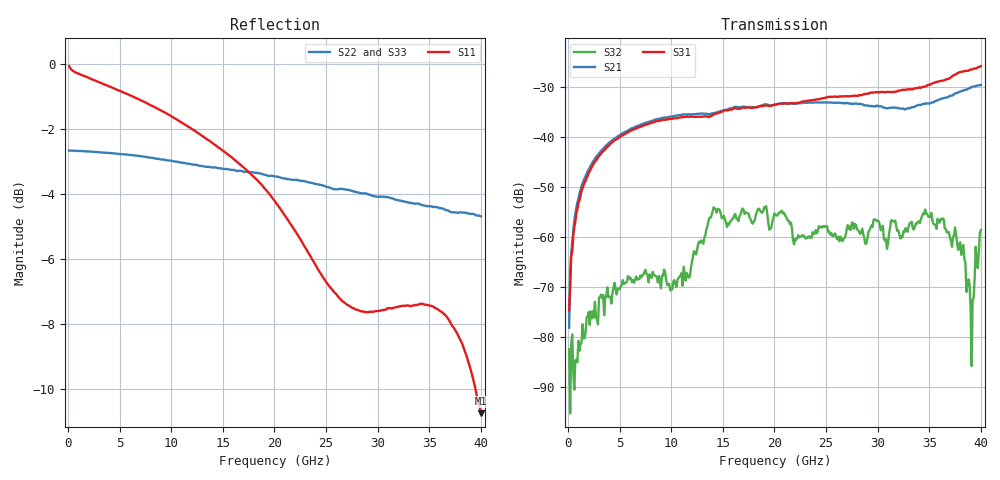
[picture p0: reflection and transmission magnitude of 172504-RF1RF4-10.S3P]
!  3-Port S-parameters saved by WinCal
! VAR MeasName=S-Parameters (CALIBRATED_DATA) read from VNA (N5245A)
! VAR MeasDate=2017-3-15 11:11:30
! VAR NAME=172504-RF1RF4-10
! VAR FILENAME=172504-RF1RF4-10.S3P
! VAR DATE=2017-3-15 11:11:30
! VAR PHYS_PORTS=1,2,3
# Hz S DB R 50
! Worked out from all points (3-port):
!   400 points, 100 MHz to 40 GHz, reference 50 ohm
!   strongest paths, dB at 100 MHz, 10.1 GHz, 20.1 GHz, 30.1 GHz, 40 GHz:
!     S31: -74.8, -36.4, -33.5, -31.1, -25.8
!     S21: -78.2, -35.8, -33.4, -33.9, -29.6
!     S32: -82.5, -70.5, -55.6, -56.9, -58.7
!   lowest |S11| = -10.8 dB at 40 GHz (marker M1), VSWR 1.82, Z = 29.5 - j11.1 ohm
!   |S11| at or under -10 dB: 39.47 GHz to end of sweep
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1e8  -0.07 -2.0  -74.94 93.4  -78.59 131.4
     -78.20 112.2  -2.66 179.8  -89.74 -169.0
     -74.77 78.0  -82.53 23.4  -2.63 179.8
8e8  -0.27 -12.3  -54.13 90.6  -55.63 94.5
     -54.14 90.9  -2.67 178.3  -84.94 83.9
     -55.31 95.2  -84.57 66.1  -2.64 178.3
3.2e9  -0.59 -45.5  -42.85 64.8  -43.36 69.0
       -42.77 65.1  -2.72 173.2  -70.72 77.9
       -43.28 68.8  -71.58 81.7  -2.69 173.4
1.19e10  -1.98 -140.3  -35.48 12.5  -35.96 17.4
         -35.50 12.4  -3.08 155.5  -66.66 118.5
         -35.95 17.6  -66.24 121.4  -3.02 155.8
2.01e10  -4.25 139.4  -33.46 -17.6  -33.49 -7.1
         -33.45 -17.2  -3.46 137.8  -55.50 36.9
         -33.54 -6.9  -55.64 37.6  -3.39 138.3
2.82e10  -7.58 14.7  -33.22 -55.8  -31.40 -39.0
         -33.34 -54.7  -3.96 117.9  -58.05 25.5
         -31.62 -37.9  -59.00 30.8  -3.91 118.2
3.63e10  -7.66 -93.6  -31.94 -72.2  -28.26 -71.6
         -32.28 -69.1  -4.45 94.6  -55.56 8.6
         -28.73 -68.6  -56.32 7.6  -4.54 94.3
3.83e10  -8.71 -118.7  -30.37 -80.0  -26.64 -84.4
         -30.69 -76.9  -4.57 88.5  -62.56 -34.5
         -26.84 -80.7  -61.61 -36.8  -4.70 87.9
3.91e10  -9.51 -130.0  -29.72 -85.3  -26.21 -91.2
         -30.04 -81.4  -4.61 85.8  -74.87 -179.5
         -26.47 -87.2  -85.88 -4.5  -4.76 85.5
4e10  -10.75 -143.7  -29.27 -90.5  -25.65 -97.8
      -29.60 -86.4  -4.69 82.6  -58.61 144.3
      -25.82 -92.3  -58.66 148.4  -4.81 82.8
